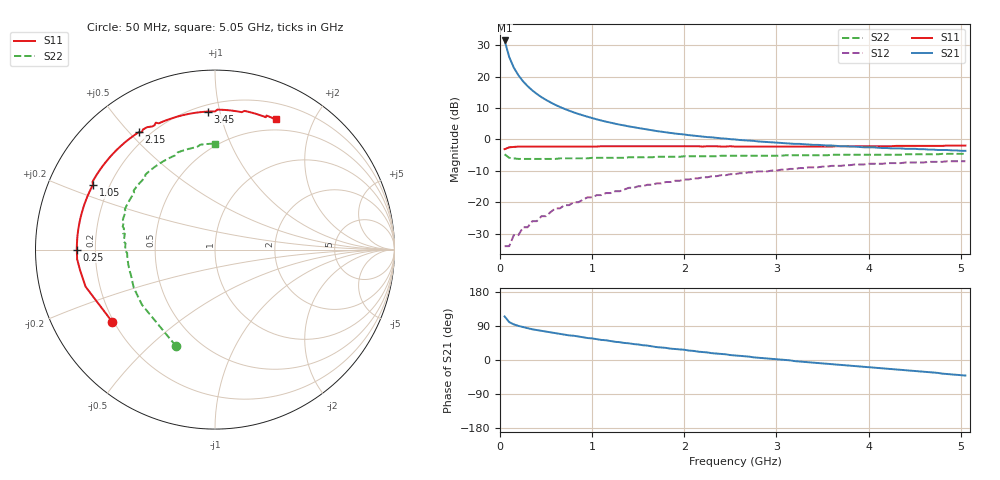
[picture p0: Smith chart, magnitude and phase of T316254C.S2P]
!AT-31625
!S-PARAMETERS at Vce=3.6 V  Ic=150 mA.  LAST UPDATED 08-05-96
# ghz s ma r 50
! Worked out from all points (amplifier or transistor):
!   101 points, 50 MHz to 5.05 GHz, reference 50 ohm
!   highest |S21| = 31.5 dB at 50 MHz (marker M1)
!   |S21| within 3 dB of that: start of sweep to 78.43 MHz
!   unconditionally stable (mu >= 1): 393.2 MHz to 427.2 MHz; 457.5 MHz to 1.395 GHz; 1.405 GHz to 1.482 GHz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
!   at 850 MHz: K = 1.06, MAG = 12.6 dB, |S12| = -20.0 dB
!   at 2.55 GHz: K = 0.98, MSG = 5.5 dB, |S12| = -11.1 dB
!   at 5.05 GHz: K = 0.95, MSG = 1.7 dB, |S12| = -6.9 dB
!   S11 on the Smith chart (normalised r, x): 50 MHz: 0.19, -0.30; 250 MHz: 0.13, -0.00; 1.05 GHz: 0.14, +0.24; 2.15 GHz: 0.16, +0.53; 3.45 GHz: 0.24, +0.92; 5.05 GHz: 0.37, +1.50
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0.05  0.7 -145.0  37.67 115.0  0.02 42.0  0.58 -112.0
0.1  0.75 -164.0  20.52 100.0  0.02 43.0  0.51 -143.0
0.15  0.76 -171.0  13.89 94.0  0.03 48.0  0.5 -155.0
0.2  0.77 -176.0  10.49 90.0  0.03 53.0  0.49 -162.0
0.25  0.77 -180.0  8.43 87.0  0.04 56.0  0.49 -166.0
0.3  0.77 178.0  7.04 84.0  0.04 59.0  0.49 -169.0
0.35  0.77 175.0  6.05 81.0  0.05 61.0  0.49 -171.0
0.4  0.77 173.0  5.3 79.0  0.05 62.0  0.49 -173.0
0.45  0.77 171.0  4.72 77.0  0.06 63.0  0.49 -175.0
0.55  0.77 168.0  3.88 73.0  0.07 64.0  0.49 -177.0
0.65  0.77 164.0  3.29 69.0  0.08 64.0  0.5 -179.0
0.75  0.77 161.0  2.87 65.0  0.09 63.0  0.5 179.0
0.9  0.77 157.0  2.42 60.0  0.11 62.0  0.5 177.0
1.05  0.77 152.0  2.09 55.0  0.13 60.0  0.51 175.0
1.35  0.78 144.0  1.67 45.0  0.16 56.0  0.51 170.0
1.75  0.78 134.0  1.33 33.0  0.2 50.0  0.53 165.0
2.15  0.78 123.0  1.13 22.0  0.24 43.0  0.54 160.0
2.55  0.77 114.0  1 12.0  0.28 36.0  0.55 153.0
3.4  0.77 94.0  0.82 -7.0  0.36 20.0  0.56 138.0
3.45  0.77 93.0  0.82 -8.0  0.36 19.0  0.56 137.0
4.25  0.78 79.0  0.72 -24.0  0.42 2.0  0.57 115.0
5.05  0.8 65.0  0.66 -41.0  0.45 -14.0  0.59 90.0
